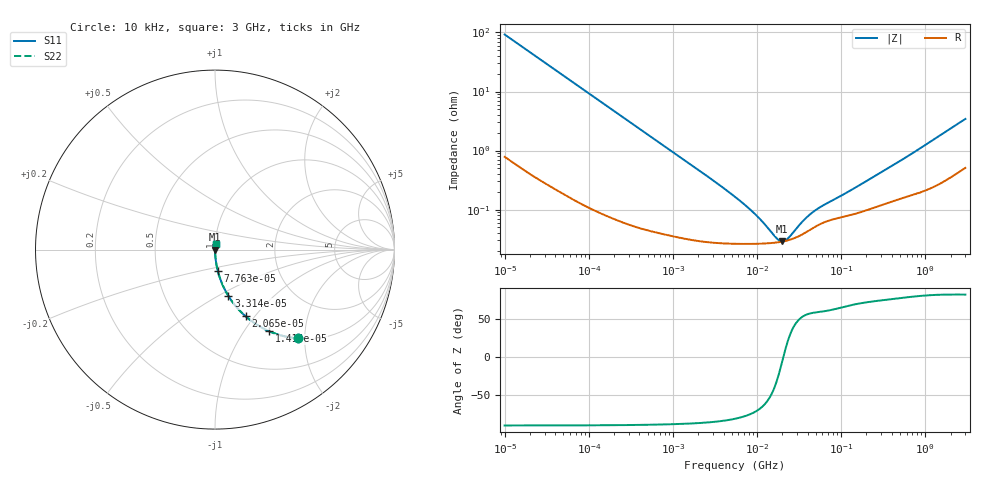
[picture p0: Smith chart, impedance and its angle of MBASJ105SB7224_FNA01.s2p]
! MBASJ105SB7224_FNA01  S-PARAMETER MODEL  ( Standard Model )
! Model Generated by TAIYO YUDEN Corporation (http://www.ty-top.com)
! Version 2.0
! TAIYO YUDEN Control No. 230609
! Copyright(c) 2013 TAIYO YUDEN CO.,LTD. All Rights Reserved.
! Product Description (link to TY-COMPAS)
! https://ds.yuden.co.jp/TYCOMPAS/or/detail?pn=MBASJ105SB7224KFNA01&u=M
! Products Name : Multilayer Ceramic Capacitors
! Characteristics :
!  Capacitance : 0.22 [uF] , Rated Voltage : 6.3 [V] , TCC : X7R
!  Case Size : 1.0 x 0.5 / 0.039 x 0.02 [mm/inch] , Thickness : 0.5 / 0.02 [mm/inch]
!  (Conditions: Temperature = 25 [degC] , DC Bias Voltage = 0 [V])
! External Node Assignments :
!  1  o---| |---o  2
! GND o---------o GND
! Frequency Range : 10kHz  -  3GHz  [ 401 STEP ]
# MHZ S RI R 50
! Freq[MHz].  S11 Real  S11 Imag  S21 Real  S21 Imag  S12 Real  S12 Imag  S22 Real  S22 Imag
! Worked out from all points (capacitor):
!   401 points, 10 kHz to 3 GHz, reference 50 ohm
!   read as one part in series: C = 172 nF near 10.65 kHz
!   lowest |Z| = 28.9 mohm at 19.95 MHz (marker M1)
!   series resonance near 20.57 MHz, so ESL is about 350 pH
!   S11 on the Smith chart (normalised r, x): 10 kHz: 1.02, -1.85; 14.15 kHz: 1.01, -1.31; 20.65 kHz: 1.01, -0.90; 33.14 kHz: 1.01, -0.56; 77.63 kHz: 1.00, -0.24; 3 GHz: 1.01, +0.07
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0.01  0.4609 -0.4942  0.5391 0.4942  0.5391 0.4942  0.4609 -0.4942
0.014146  0.3014 -0.4546  0.6986 0.4546  0.6986 0.4546  0.3014 -0.4546
0.020651  0.17 -0.3713  0.83 0.3713  0.83 0.3713  0.17 -0.3713
0.033138  0.075 -0.2588  0.925 0.2588  0.925 0.2588  0.075 -0.2588
0.049927  0.0353 -0.1797  0.9647 0.1797  0.9647 0.1797  0.0353 -0.1797
0.07763  0.0155 -0.1183  0.9845 0.1183  0.9845 0.1183  0.0155 -0.1183
0.082683  0.0138 -0.1113  0.9862 0.1113  0.9862 0.1113  0.0138 -0.1113
0.199902  0.00289 -0.0468  0.9971 0.0468  0.9971 0.0468  0.00289 -0.0468
0.683653  0.00059 -0.0138  0.9994 0.0138  0.9994 0.0138  0.00059 -0.0138
2.570001  0.000294 -0.00366  0.9997 0.00366  0.9997 0.00366  0.000294 -0.00366
5.477226  0.000266 -0.00163  0.9997 0.00163  0.9997 0.00163  0.000266 -0.00163
9.97066  0.000264 -0.000737  0.9997 0.000737  0.9997 0.000737  0.000264 -0.000737
17.04125  0.000277 -0.000178  0.9997 0.000178  0.9997 0.000178  0.000277 -0.000178
19.95104  0.000287 -2.88e-05  0.9997 2.88e-05  0.9997 2.88e-05  0.000287 -2.88e-05
21.24962  0.000292 3.03e-05  0.9997 -3.03e-05  0.9997 -3.03e-05  0.000292 3.03e-05
23.35767  0.000302 0.000119  0.9997 -0.000119  0.9997 -0.000119  0.000302 0.000119
35.19136  0.000386 0.000511  0.9996 -0.000511  0.9996 -0.000511  0.000386 0.000511
45.28751  0.000479 0.000749  0.9995 -0.000749  0.9995 -0.000749  0.000479 0.000749
60.14696  0.000594 0.001  0.9994 -0.001  0.9994 -0.001  0.000594 0.001
124.2076  0.0008 0.00188  0.9992 -0.00188  0.9992 -0.00188  0.0008 0.00188
374.4521  0.00135 0.005  0.9986 -0.005  0.9986 -0.005  0.00135 0.005
3000  0.00619 0.0336  0.9938 -0.0336  0.9938 -0.0336  0.00619 0.0336
